(* Logix 5000 AddOnInstructionDefinition export AOI_UDDT_Compare; software revision 36.00 *)

TYPE DUT_NDSN_spLink_Bead :
STRUCT
   di_rw_NumOfBeads : DINT;
   di_rw_BeadDelay : DINT[8];   // 1/4 mm
   di_rw_BeadDuration : DINT[8];   // 1/4 mm
   di_rw_mode : DINT;   // 1/4 mm
   di_rw_MaxGunTime : DINT;   // microseconds
   di_rw_LineSpeedActivation : DINT;   // 100th m/min
   di_rw_LineSpeedDeactivation : DINT;   // 100th m/min
   di_rw_Interval : DINT;   // 1/4 mm
   di_rw_AdhesiveSavings : DINT;   // 30%-60%
   di_rw_EcoBeadPattern : DINT;   // 0-40, Illegal values: 0,1,11,20,21,30,31,38,39
END_STRUCT
END_TYPE

ADD_ON_INSTRUCTION AOI_UDDT_Compare   (* revision 1.0 *)
VAR_INPUT
   UDDT_INT_SIZE : DINT; {access Read Only, required}
END_VAR
VAR_IN_OUT
   UDDT_1 : DUT_NDSN_spLink_Bead; {required}
   UDDT_2 : DUT_NDSN_spLink_Bead; {required}
END_VAR
VAR_OUTPUT
   NOT_EQUAL : BOOL; {visible}
   EQUAL : BOOL; {visible}
END_VAR
VAR_INPUT
   i_count : INT; {access Read Only}
END_VAR
VAR
   i_buffer1 : DINT[100]; {access None}
   i_buffer2 : DINT[100]; {access None}
   d_count : INT; {access None}
   d_size : INT; {access None}
END_VAR

ROUTINE Logic   (* structured text *)
   //****************************************************************************************************
   //*****  UDDT Compare
   //*****
   //*****  DESCRIPTION:  Subroutine to compare to UDDTs of equal length.  If a difference is located, the NOT_EQUAL output
   //*****					Bit is set.  Otherwise, the EQUAL Bit is set.
   //*****
   //*****
   
   EQUAL := 1;
   NOT_EQUAL := 0;
   i_count := 0;
   d_size := UDDT_INT_SIZE/2;
   
   COP(UDDT_1.di_rw_NumOfBeads, i_buffer1[0], d_size);
   COP(UDDT_2.di_rw_NumOfBeads, i_buffer2[0], d_size);
   
   
   FOR i_count :=0 TO d_size-1 BY 1 DO
   	IF (i_buffer1[i_count] <> i_buffer2[i_count])  THEN
   
   		EQUAL := 0;
   		NOT_EQUAL := 1;
   		EXIT;
   	END_IF;
   END_FOR;
   
END_ROUTINE
END_ADD_ON_INSTRUCTION
